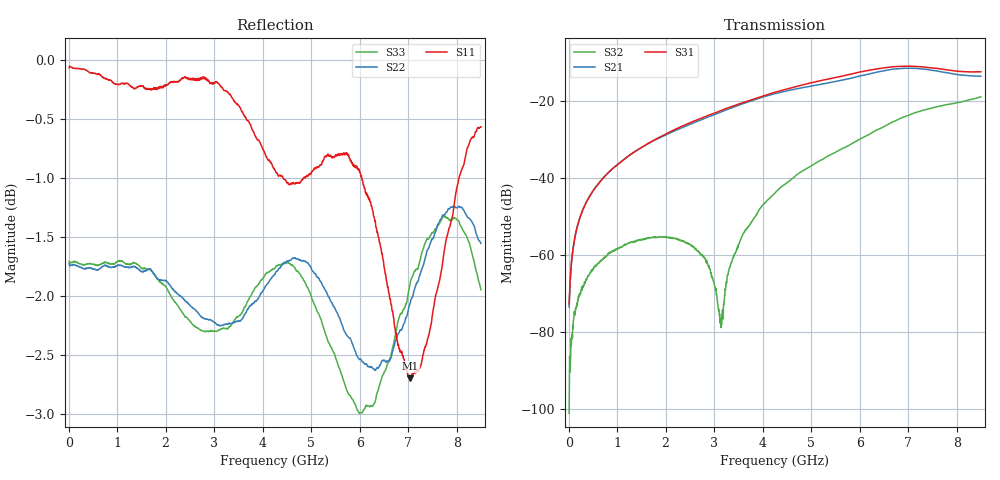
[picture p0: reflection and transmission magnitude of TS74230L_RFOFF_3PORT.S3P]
!Agilent Technologies,E5071C,MY46522130,B.12.04
!Date: Fri Aug 01 10:38:15 2025
!Data & Calibration Information:
!Freq	S11:SOLT3(ON)	S13:SOLT3(ON)	S14:SOLT3(ON)
!	S31:SOLT3(ON)	S33:SOLT3(ON)	S34:SOLT3(ON)
!	S41:SOLT3(ON)	S43:SOLT3(ON)	S44:SOLT3(ON)
!PortZ  Port1:50+j0  Port3:50+j0  Port4:50+j0
!Above PortZ is port z conversion or system Z0 setting when saving the data.
!When reading, reference impedance value at option line is always used.
# Hz S dB R 50
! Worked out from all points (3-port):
!   1601 points, 10 MHz to 8.5 GHz, reference 50 ohm
!   strongest paths, dB at 10 MHz, 2.132 GHz, 4.255 GHz, 6.378 GHz, 8.5 GHz:
!     S31: -72.7, -27.8, -17.8, -11.7, -12.5
!     S21: -73.5, -28.1, -18.1, -12.5, -13.6
!     S32: -101.1, -55.8, -43.9, -27.4, -19.0
!   lowest |S11| = -2.7 dB at 7.046 GHz (marker M1), VSWR 6.49, Z = 11.7 + j35.3 ohm
!   |S11| at or under -10 dB: nowhere
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1e7  -0.06 -0.3  -73.36 38.5  -73.55 42.1
     -73.54 43.5  -1.72 179.4  -97.13 106.1
     -72.68 37.4  -101.11 119.9  -1.70 179.4
3.9205e8  -0.09 -12.4  -45.62 89.3  -45.72 89.8
          -45.57 89.6  -1.76 170.9  -65.58 82.7
          -45.72 89.9  -65.50 84.5  -1.73 170.7
1.75045e9  -0.24 -59.6  -30.41 84.4  -30.28 85.9
           -30.41 84.4  -1.81 141.6  -55.43 60.3
           -30.28 85.9  -55.47 59.4  -1.81 142.7
2.779862e9  -0.15 -82.9  -24.70 72.1  -24.28 71.7
            -24.71 72.0  -2.19 115.6  -60.39 36.7
            -24.30 71.7  -60.27 35.2  -2.30 112.2
3.145994e9  -0.23 -89.8  -22.86 66.5  -22.51 65.8
            -22.87 66.4  -2.25 105.1  -79.14 -38.8
            -22.51 65.7  -77.02 -32.2  -2.28 100.7
3.570494e9  -0.44 -99.9  -20.85 57.9  -20.56 57.1
            -20.86 57.8  -2.20 91.6  -55.37 -150.2
            -20.56 56.9  -55.29 -150.9  -2.14 87.1
4.255e9  -0.93 -125.8  -18.13 40.3  -17.77 41.0
         -18.14 40.1  -1.81 73.0  -43.98 -174.3
         -17.79 40.9  -43.92 -174.3  -1.76 73.1
5.974225e9  -0.93 175.0  -13.68 -5.0  -12.62 -8.2
            -13.65 -4.9  -2.52 31.4  -30.09 133.9
            -12.61 -8.1  -30.15 134.0  -2.98 21.4
7.046088e9  -2.70 107.6  -11.51 -48.9  -11.02 -52.0
            -11.55 -48.9  -2.05 -3.5  -23.65 95.4
            -11.03 -52.0  -23.57 95.5  -1.88 -13.0
8.5e9  -0.57 36.3  -13.60 -95.5  -12.44 -97.5
       -13.62 -95.7  -1.55 -30.0  -19.06 42.1
       -12.47 -97.7  -18.96 41.7  -1.95 -34.3
